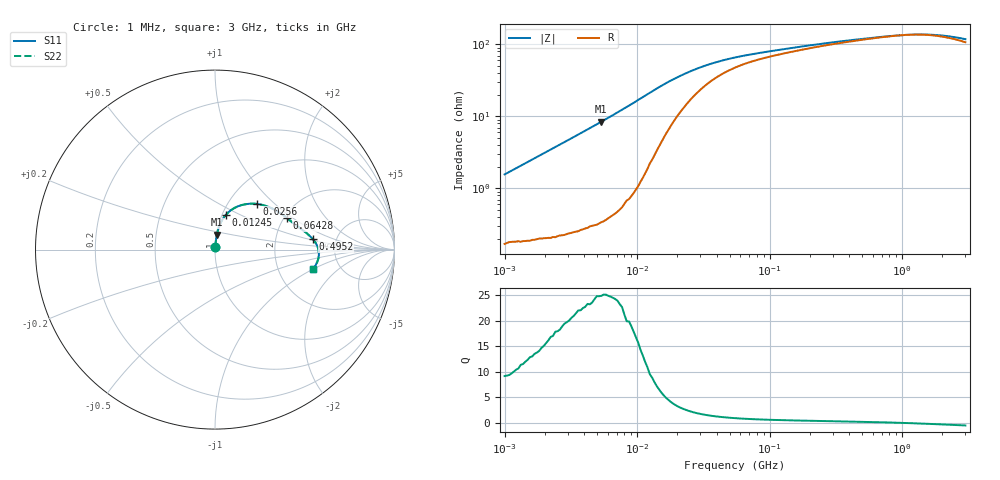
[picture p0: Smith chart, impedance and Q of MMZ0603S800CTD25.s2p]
! S-Parameter Data Generated by TDK Corporation
! Copyright(C) 2025 TDK Corporation.
! All Rights Reserved.
! TDK P/N: MMZ0603S800CTD25 (Chip Bead)
! Property: |Z|=80ohm at 100MHz
! Size(LxWxT): 0.6x0.3x0.3mm
! Model Type: s2p (Touchstone File Format Version 1.0)
! Frequency: DC=Yes Start=1MHz Stop=3000MHz 202points Log-sweep
! Model Generated on Feb. 6, 2025
! Terms and conditions regarding TDK Simulation Models:
! 1)This simulation model is being provided solely for informational
!  purposes. Please refer to the specifications of the products in
!  terms of detailed characteristics of such products.
! 2)In no event shall TDK Corporation of any of its subsidiaries be
!  liable for any loss or damage arising, directly or indirectly,
!  from any information contained in this simulation model, including,
!  but not limited to loss or damages arising from any inaccuracies,
!  omissions or errors in connection with such information.
! 3)Any and all copyrights on this simulation model are owned by
!  TDK Corporation.  Duplication or redistribution of this simulation
!  model without prior written permission from TDK Corporation
!  is prohibited.
! 4)This simulation model is subject to any modification or change
!  without any prior notice.
! 5)Neither TDK Corporation nor any of its subsidiaries shall make any
!  warranty, express or implied, including but not limited to the
!  correctness, implied warranties of merchantability and fitness for
!  a particular purpose with respect to this simulation models.
! 6)The use of this simulation model shall be deemed to have consented
!  to the terms and conditions hereof.
! Port Assignments:
!  1 ---@@@--- 2
! Applicable Conditions:
!  Temperature = 25 degC
!  DC Bias Current = 0 A
!  Small Signal Operation
# Hz S MA R 50
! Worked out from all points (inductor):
!   201 points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, 1 MHz to 3 GHz, reference 50 ohm
!   read as one part in series: L = 248 nH near 1.041 MHz
!   highest Q = 24.8 at 5.373 MHz (marker M1), where L = 250 nH
!   self-resonance near 1.112 GHz
!   S11 on the Smith chart (normalised r, x): 1 MHz: 1.00, +0.03; 12.45 MHz: 1.04, +0.42; 25.6 MHz: 1.35, +0.78; 64.28 MHz: 2.07, +0.90; 495.2 MHz: 3.31, +0.56; 3 GHz: 3.14, -1.00
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1000000  0.01566 82.9  0.9982 -0.9  0.9982 -0.9  0.01566 82.9
2055611  0.03193 84.5  0.9974 -1.8  0.9974 -1.8  0.03193 84.5
3900413  0.06064 84.0  0.9955 -3.5  0.9955 -3.5  0.06064 84.0
5372736  0.08396 82.9  0.9931 -4.8  0.9931 -4.8  0.08396 82.9
7110411  0.1125 81.1  0.989 -6.5  0.989 -6.5  0.1125 81.1
9040831  0.1452 78.6  0.9818 -8.3  0.9818 -8.3  0.1452 78.6
1.245355e7  0.2046 72.3  0.9578 -11.7  0.9578 -11.7  0.2046 72.3
1.461624e7  0.2385 67.7  0.936 -13.6  0.936 -13.6  0.2385 67.7
1.71545e7  0.2726 62.2  0.9054 -15.4  0.9054 -15.4  0.2726 62.2
1.934349e7  0.2966 57.7  0.878 -16.6  0.878 -16.6  0.2966 57.7
2.559965e7  0.3456 47.4  0.8071 -18.4  0.8071 -18.4  0.3456 47.4
3.670325e7  0.392 35.8  0.7198 -18.6  0.7198 -18.6  0.392 35.8
5.477226e7  0.4263 26.6  0.6474 -17.1  0.6474 -17.1  0.4263 26.6
6.428402e7  0.4371 23.8  0.6253 -16.4  0.6253 -16.4  0.4371 23.8
1.039275e8  0.4656 17.7  0.5742 -14.3  0.5742 -14.3  0.4656 17.7
2.136344e8  0.5067 11.8  0.5145 -11.6  0.5145 -11.6  0.5067 11.8
4.951867e8  0.5473 6.2  0.4598 -7.4  0.4598 -7.4  0.5473 6.2
8.005644e8  0.5666 2.8  0.435 -3.7  0.435 -3.7  0.5666 2.8
1.147801e9  0.577 -0.3  0.423 0.4  0.423 0.4  0.577 -0.3
1.581072e9  0.5792 -3.7  0.4236 5.0  0.4236 5.0  0.5792 -3.7
2.092429e9  0.5738 -6.9  0.4358 9.1  0.4358 9.1  0.5738 -6.9
3e9  0.5547 -11.4  0.4693 13.5  0.4693 13.5  0.5547 -11.4
